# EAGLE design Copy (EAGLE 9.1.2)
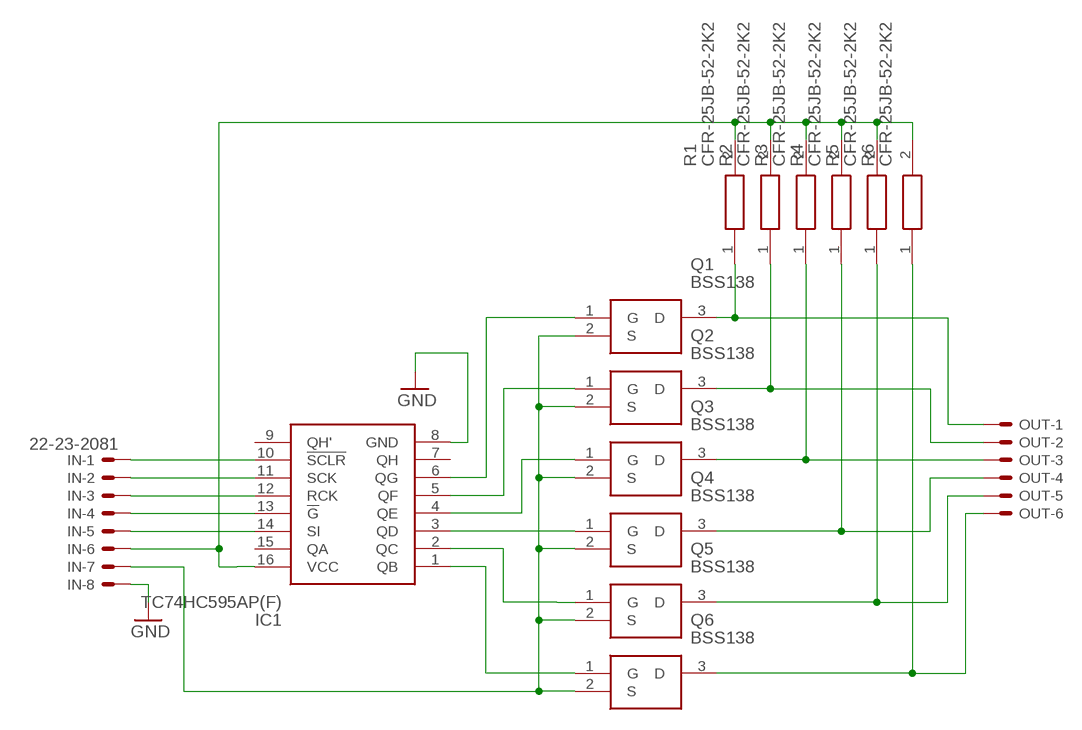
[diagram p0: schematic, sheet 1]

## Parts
IC1  TC74HC595AP(F)  [DIP762W60P254L1925H445Q16N]
IN  22-23-2081  [22-23-2081]
OUT  22-23-2061  [22-23-2061]
Q1  BSS138  [SOT95P240X120-3N]
Q2  BSS138  [SOT95P240X120-3N]
Q3  BSS138  [SOT95P240X120-3N]
Q4  BSS138  [SOT95P240X120-3N]
Q5  BSS138  [SOT95P240X120-3N]
Q6  BSS138  [SOT95P240X120-3N]
R1  CFR-25JB-52-2K2  [RESAD1590W60L630D240]
R2  CFR-25JB-52-2K2  [RESAD1590W60L630D240]
R3  CFR-25JB-52-2K2  [RESAD1590W60L630D240]
R4  CFR-25JB-52-2K2  [RESAD1590W60L630D240]
R5  CFR-25JB-52-2K2  [RESAD1590W60L630D240]
R6  CFR-25JB-52-2K2  [RESAD1590W60L630D240]

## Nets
GND: IC1.8(GND) IN.8
N$1: IN.7 Q1.2(S) Q2.2(S) Q3.2(S) Q4.2(S) Q5.2(S) Q6.2(S)
N$2: IC1.1(QB) Q6.1(G)
N$3: IC1.3(QD) Q4.1(G)
N$4: IC1.2(QC) Q5.1(G)
N$5: IC1.6(QG) Q1.1(G)
N$6: IC1.5(QF) Q2.1(G)
N$7: IC1.4(QE) Q3.1(G)
N$8: IC1.10(!SCLR) IN.1
N$9: IC1.11(SCK) IN.2
N$10: IC1.12(RCK) IN.3
N$11: IC1.13(!G) IN.4
N$12: IC1.14(SI) IN.5
N$13: IC1.16(VCC) IN.6 R1.2 R2.2 R3.2 R4.2 R5.2 R6.2
N$14: OUT.1 Q1.3(D) R1.1
N$15: OUT.2 Q2.3(D) R2.1
N$16: OUT.3 Q3.3(D) R3.1
N$17: OUT.4 Q4.3(D) R4.1
N$18: OUT.5 Q5.3(D) R5.1
N$19: OUT.6 Q6.3(D) R6.1
Unconnected: IC1.7(QH) IC1.9(QH') IC1.15(QA)

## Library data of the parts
IC1 = TC74HC595AP(F):TC74HC595AP(F): IC,CMOS logic,DIP16,SHIFT REGISTERS Source: Datasheet; DESCRIPTION: IC,CMOS logic,DIP16,SHIFT REGISTERS; HEIGHT: 4.45mm; MANUFACTURER_NAME: Toshiba; MANUFACTURER_PART_NUMBER: TC74HC595AP(F); MOUSER_PART_NUMBER: N/A; MOUSER_PRICE-STOCK: https://www.mouser.com/Search/Refine.aspx?Keyword=N%2FA; RS_PART_NUMBER: 5400095P; RS_PRICE-STOCK: http://au.rs-online.com/web/p/products/5400095P
IN = con-molex:22-23-2081: .100" (2.54mm) Center Header - 8 Pin; MF: MOLEX; MPN: 22-23-2081; OC_FARNELL: 1756826; OC_NEWARK: 01C7592
OUT = con-molex:22-23-2061: .100" (2.54mm) Center Header - 6 Pin; MF: MOLEX; MPN: 22-23-2061; OC_FARNELL: 1462922; OC_NEWARK: 27C1933
Q1-Q6 = BSS138:BSS138: N-channel MOSFET,BSS138 0.2A 50V Source: Datasheet; DESCRIPTION: N-channel MOSFET,BSS138 0.2A 50V; HEIGHT: 1.2mm; MANUFACTURER_NAME: ON Semiconductor; MANUFACTURER_PART_NUMBER: BSS138; MOUSER_PART_NUMBER: 512-BSS138; RS_PART_NUMBER: 1241694; RS_PRICE-STOCK: http://uk.rs-online.com/web/p/products/1241694
R1-R6 = CFR-25JB-52-2K2:CFR-25JB-52-2K2: Carbon Film Resistors - Through Hole 1/4W 2.2K Ohm 5%; DESCRIPTION: Carbon Film Resistors - Through Hole 1/4W 2.2K Ohm 5%; HEIGHT: mm; MANUFACTURER_NAME: YAGEO (PHYCOMP); MANUFACTURER_PART_NUMBER: CFR-25JB-52-2K2; MOUSER_PART_NUMBER: 603-CFR-25JB-52-2K2; MOUSER_PRICE-STOCK: https://www.mouser.com/Search/Refine.aspx?Keyword=603-CFR-25JB-52-2K2; RS_PART_NUMBER: 603-CFR-25JB-52-2K2; RS_PRICE-STOCK: https://www.mouser.com/Search/Refine.aspx?Keyword=603-CFR-25JB-52-2K2

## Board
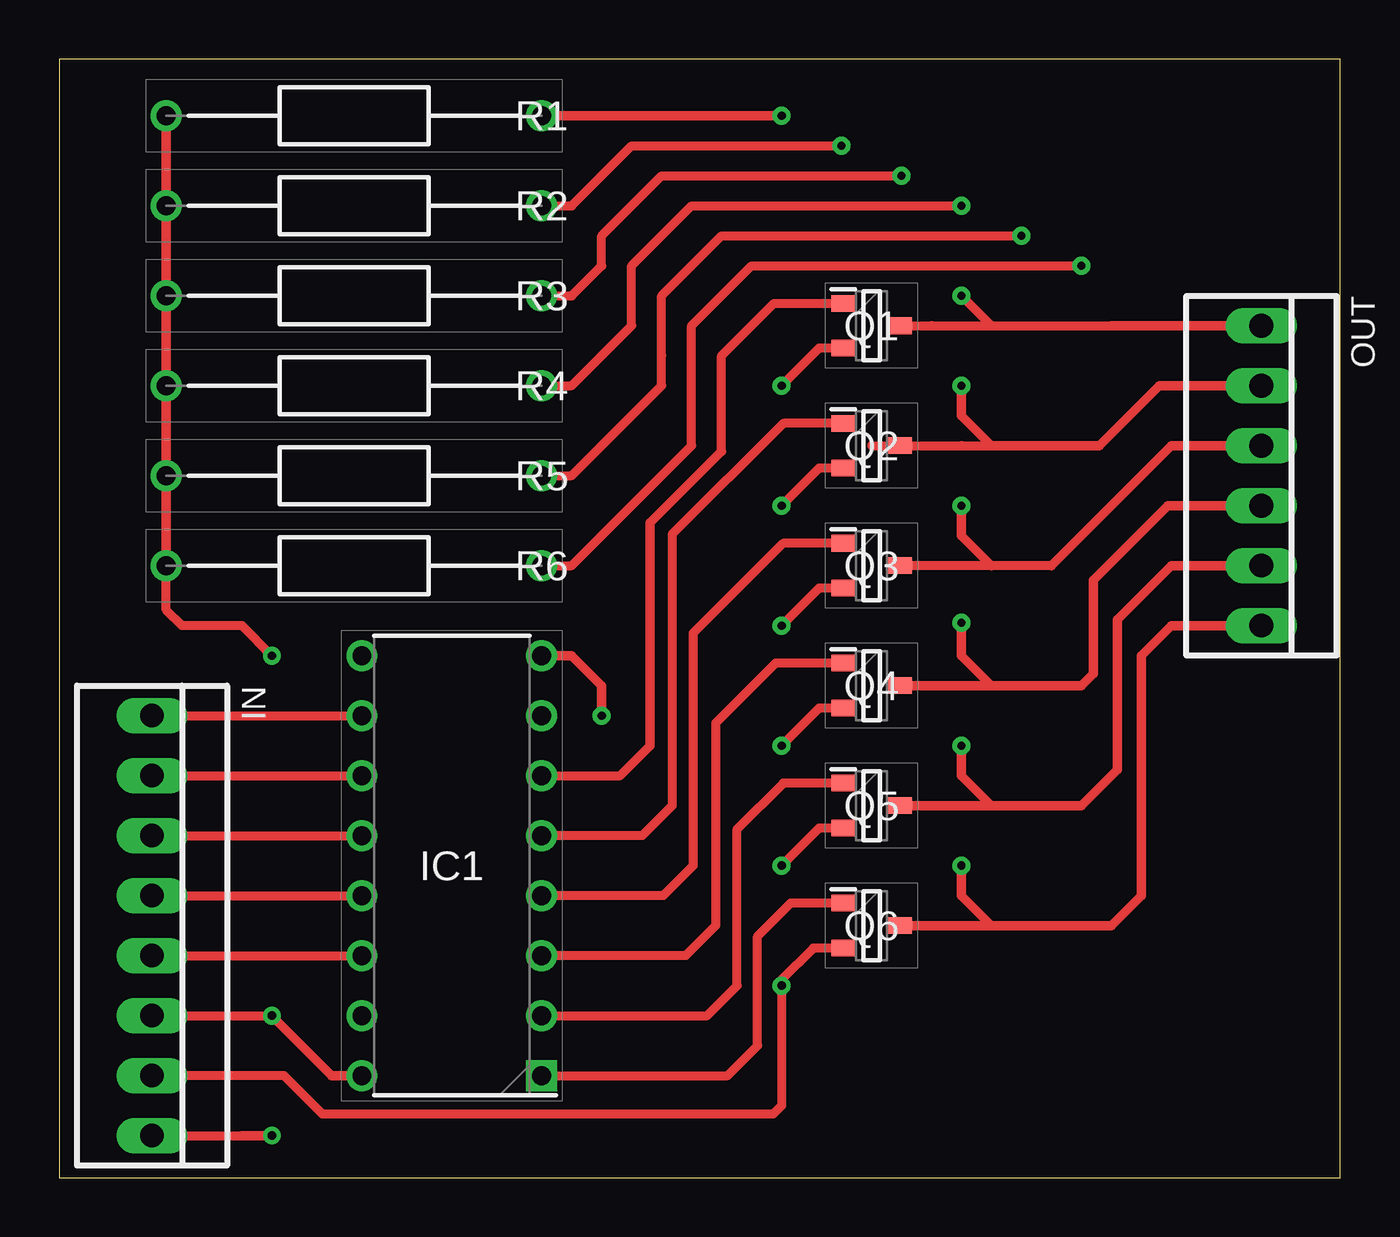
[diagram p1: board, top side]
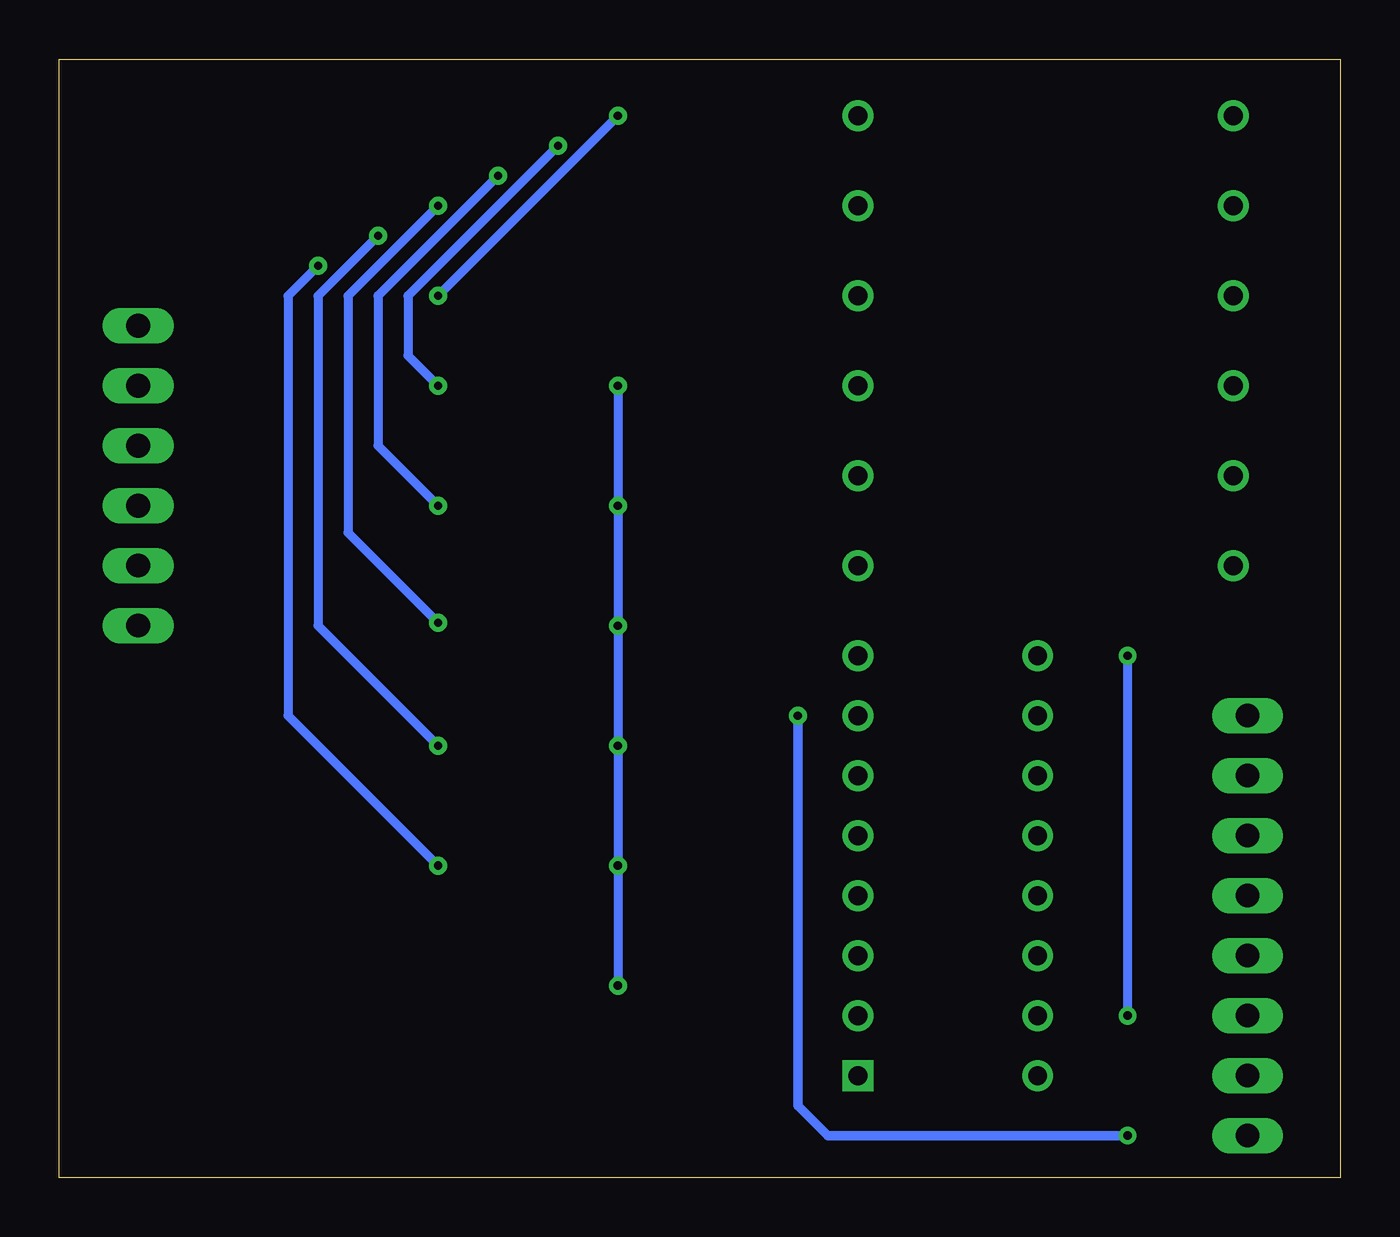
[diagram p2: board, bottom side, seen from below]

Size 54.28 x 47.36 mm. Coordinates in mm from the lower left corner, seen from the top.
Outline: 0,0 54.28,0 54.28,47.36 0,47.36 0,0
Copper layers (1*16): Top 0.035mm / dielectric 1.5mm / Bottom 0.035mm
Design rules "default": minimum track width 6mil, minimum drill 0.35mm, track to track 6mil, track to pad 6mil, pad to pad 6mil, via to via 6mil, smd to smd 6mil, copper to edge 40mil, drill to drill 6mil, minimum pad ring 10mil, minimum via ring 8mil, stop-mask expansion 4mil, vias tented up to drill 0mil, thermal gap 10mil

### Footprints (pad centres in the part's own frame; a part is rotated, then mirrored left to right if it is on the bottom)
DIP762W60P254L1925H445Q16N = drill 0.8 pad 1.2 square: 1 -3.81,8.89 | drill 0.8 pad 1.2: 2 -3.81,6.35; 3 -3.81,3.81; 4 -3.81,1.27; 5 -3.81,-1.27; 6 -3.81,-3.81; 7 -3.81,-6.35; 8 -3.81,-8.89; 9 3.81,-8.89; 10 3.81,-6.35; 11 3.81,-3.81; 12 3.81,-1.27; 13 3.81,1.27; 14 3.81,3.81; 15 3.81,6.35; 16 3.81,8.89
22-23-2081 = drill 1 long: 1 -8.89,0; 2 -6.35,0; 3 -3.81,0; 4 -1.27,0; 5 1.27,0; 6 3.81,0; 7 6.35,0; 8 8.89,0
22-23-2061 = drill 1 long: 1 -6.35,0; 2 -3.81,0; 3 -1.27,0; 4 1.27,0; 5 3.81,0; 6 6.35,0
SOT95P240X120-3N = smd 1 x 0.7: 1 -1.2,0.95; 2 -1.2,-0.95; 3 1.2,0
RESAD1590W60L630D240 = drill 0.8 pad 1.2: 1 0,0; 2 15.9,0

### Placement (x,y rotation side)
IC1  16.64,13.21 180 top
IN  3.94,10.67 270 top
OUT  50.93,29.72 270 top
Q1  34.42,36.07 0 top
Q2  34.42,30.99 0 top
Q3  34.42,25.91 0 top
Q4  34.42,20.83 0 top
Q5  34.42,15.75 0 top
Q6  34.42,10.67 0 top
R1  20.45,44.96 180 top
R2  20.45,41.15 180 top
R3  20.45,37.34 180 top
R4  20.45,33.53 180 top
R5  20.45,29.72 180 top
R6  20.45,25.91 180 top

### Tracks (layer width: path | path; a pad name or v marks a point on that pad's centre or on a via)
GND  (via drill 0.35)
  Top 0.381: IN.8 7.75,1.78
  Top 0.406: 7.75,1.78 v9.02,1.78 | IC1.8 21.72,22.1 22.99,20.83 v22.99,19.56
  Bottom 0.406: v9.02,1.78 21.72,1.78 22.99,3.05 v22.99,19.56
N$1  (via drill 0.35)
  Top 0.381: IN.7 9.53,4.32 11.17,2.69 30.24,2.69 30.61,3.05 v30.61,8.13 30.61,8.38 31.95,9.72 Q6.2 | Q2.2 32.2,30.04 v30.61,28.45 | Q3.2 32.2,24.96 v30.61,23.37 | Q4.2 32.2,19.88 v30.61,18.29 | Q5.2 32.2,14.8 v30.61,13.21 | Q1.2 32.2,35.12 v30.61,33.53
  Bottom 0.381: v30.61,33.53 v30.61,28.45 v30.61,23.37 v30.61,18.29 v30.61,13.21 v30.61,8.13
N$2
  Top 0.381: Q6.1 30.99,11.62 29.59,10.22 29.59,5.59 28.32,4.32 IC1.1
N$3
  Top 0.381: Q4.1 30.35,21.78 27.81,19.24 27.81,10.67 26.54,9.4 IC1.3
N$4
  Top 0.381: Q5.1 30.68,16.7 28.73,14.75 28.73,8.13 27.46,6.86 IC1.2
N$5
  Top 0.381: 25.04,18.29 23.77,17.02 IC1.6 | 25.04,27.72 28.07,30.74 28.07,34.8 30.29,37.02 Q1.1
  Top 0.406: 25.04,18.29 25.04,24.64 25.04,27.72
N$6
  Top 0.381: Q2.1 30.68,31.94 25.97,27.23 25.97,15.75 24.7,14.48 IC1.5
N$7
  Top 0.381: Q3.1 30.67,26.86 26.86,23.05 26.86,13.21 25.59,11.94 IC1.4
N$8
  Top 0.381: IN.1 IC1.10
N$9
  Top 0.381: IN.2 IC1.11
N$10
  Top 0.381: IN.3 IC1.12
N$11
  Top 0.381: IN.4 IC1.13
N$12
  Top 0.381: IN.5 IC1.14
N$13  (via drill 0.35)
  Top 0.381: IN.6 v9.02,6.86 | R6.2 4.55,24.03 5.21,23.37 7.75,23.37 v9.02,22.1
  Top 0.406: R6.2 R5.2 R4.2 R3.2 R2.2 R1.2 | v9.02,6.86 11.56,4.32 IC1.16
  Bottom 0.381: v9.02,6.86 v9.02,22.1
N$14  (via drill 0.35)
  Top 0.381: Q1.3 36.96,36.07 39.5,36.07 | 39.5,36.07 44.58,36.07 | v38.23,37.34 39.5,36.07
  Top 0.406: 44.58,36.07 OUT.1 | v30.61,44.96 R1.1
  Bottom 0.381: v30.61,44.96 v38.23,37.34
N$15  (via drill 0.35)
  Top 0.381: Q2.3 38.23,30.99 | 38.23,30.99 39.5,30.99 | R2.1 21.72,41.15 24.26,43.69 v33.15,43.69 | 34.42,30.99 38.23,30.99
  Top 0.406: OUT.2 46.61,33.53 44.07,30.99 39.5,30.99 38.23,32.26 v38.23,33.53
  Bottom 0.381: 39.5,37.34 39.5,34.8 v38.23,33.53
  Bottom 0.406: v33.15,43.69 39.5,37.34
N$16  (via drill 0.35)
  Top 0.381: R3.1 21.72,37.34 22.99,38.61 22.99,39.88 25.53,42.42 v35.69,42.42 | 42.04,25.91 39.5,25.91 Q3.3
  Top 0.406: OUT.3 47.12,30.99 42.04,25.91 | v38.23,28.45 38.23,27.18 39.5,25.91
  Bottom 0.381: 40.77,37.34 40.77,30.99 v38.23,28.45
  Bottom 0.406: v35.69,42.42 40.77,37.34
N$17  (via drill 0.35)
  Top 0.381: R4.1 21.72,33.53 | 35.69,20.83 Q4.3 | 29.34,41.15 30.61,41.15 | 30.61,41.15 v38.23,41.15 | 21.72,33.53 | 21.72,33.53 22.99,34.8 24.26,36.07 24.26,38.61 26.8,41.15 30.61,41.15
  Top 0.406: OUT.4 46.96,28.45 43.81,25.3 43.81,21.34 43.31,20.83 39.5,20.83 | 39.5,20.83 35.69,20.83 | v38.23,23.5 38.23,22.1 39.5,20.83
  Bottom 0.381: v38.23,41.15 42.04,37.34 42.04,27.3 v38.23,23.5
N$18  (via drill 0.35)
  Top 0.381: R5.1 21.72,29.72 25.53,33.53 25.53,34.8 25.53,37.34 28.07,39.88 v40.77,39.88
  Top 0.406: OUT.5 47.12,25.91 44.83,23.62 44.83,17.27 43.31,15.75 39.5,15.75 | 39.5,15.75 Q5.3 | v38.23,18.29 38.23,17.02 39.5,15.75
  Bottom 0.381: v38.23,18.29 43.31,23.37 43.31,37.34 v40.77,39.88
N$19  (via drill 0.35)
  Top 0.381: 20.77,25.91 R6.1 21.72,25.91 26.8,30.99 26.8,36.07 29.34,38.61 34.42,38.61 | 35.69,10.67 Q6.3 | 33.47,38.61 34.42,38.61 | 34.42,38.61 v43.31,38.61
  Top 0.406: OUT.6 47.12,23.37 45.85,22.1 45.85,11.94 44.58,10.67 43.31,10.67 39.5,10.67 | 39.5,10.67 35.69,10.67 | v38.23,13.21 38.23,11.94 39.5,10.67
  Bottom 0.381: v43.31,38.61 44.58,37.34 44.58,19.56 v38.23,13.21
